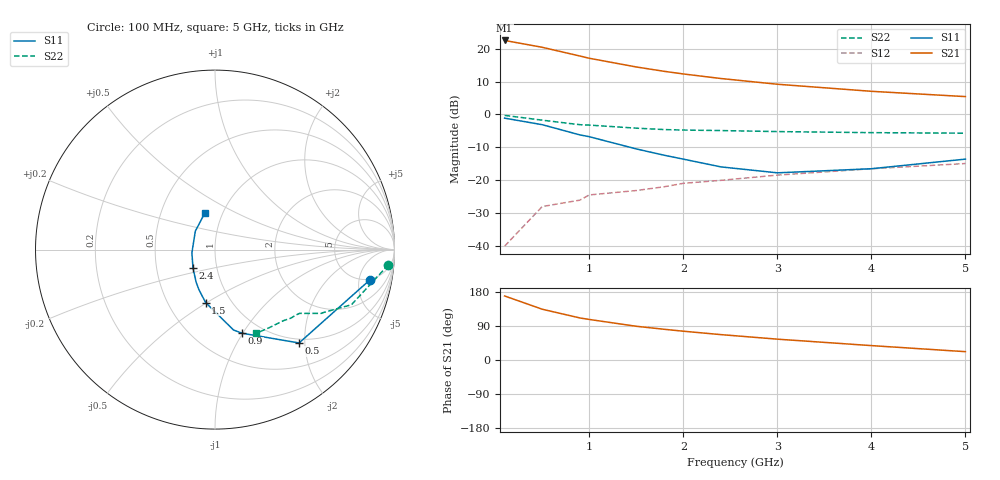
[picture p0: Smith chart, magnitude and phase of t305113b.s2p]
!AT-30511
!S and NOISE PARAMETERS at Vce=2.7V  Ic=5mA.  LAST UPDATED 04-10-94
# ghz s ma r 50
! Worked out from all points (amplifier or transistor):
!   11 points, 100 MHz to 5 GHz, reference 50 ohm
!   highest |S21| = 22.5 dB at 100 MHz (marker M1)
!   |S21| within 3 dB of that: start of sweep to 639.6 MHz
!   unconditionally stable (mu >= 1): 1.797 GHz to end of sweep
!   at 500 MHz: K = 0.43, MSG = 24.2 dB, |S12| = -28.0 dB
!   at 1.8 GHz: K = 1.00, MAG = 17.3 dB, |S12| = -21.9 dB
!   at 5 GHz: K = 1.10, MAG = 8.2 dB, |S12| = -14.9 dB
!   lowest NFmin = 1.10 dB at 500 MHz
!   S11 on the Smith chart (normalised r, x): 100 MHz: 4.83, -7.19; 500 MHz: 0.92, -1.88; 900 MHz: 0.81, -0.99; 1.5 GHz: 0.76, -0.49; 2.4 GHz: 0.77, -0.16; 5 GHz: 0.82, +0.35
0.1  0.88 -11.0  13.32 169.0  0.01 83.0  0.97 -5.0
0.5  0.7 -48.0  10.49 134.0  0.04 64.0  0.82 -22.0
0.9  0.49 -72.0  7.73 111.0  0.05 57.0  0.7 -30.0
1  0.46 -77.0  7.15 107.0  0.06 55.0  0.69 -31.0
1.5  0.3 -100.0  5.27 89.0  0.07 53.0  0.62 -35.0
1.8  0.24 -112.0  4.52 81.0  0.08 52.0  0.59 -37.0
2  0.21 -120.0  4.13 76.0  0.09 52.0  0.58 -39.0
2.4  0.16 -140.0  3.52 67.0  0.1 50.0  0.57 -42.0
3  0.13 -172.0  2.88 55.0  0.12 48.0  0.55 -46.0
4  0.15 137.0  2.25 38.0  0.15 44.0  0.53 -55.0
5  0.21 106.0  1.87 22.0  0.18 39.0  0.52 -64.0
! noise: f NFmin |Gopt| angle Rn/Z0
0.5  1.1  0.77  9  1.1
0.9  1.2  0.71  18  0.96
1.8  1.5  0.6  45  0.66
2.4  1.8  0.51  65  0.47
